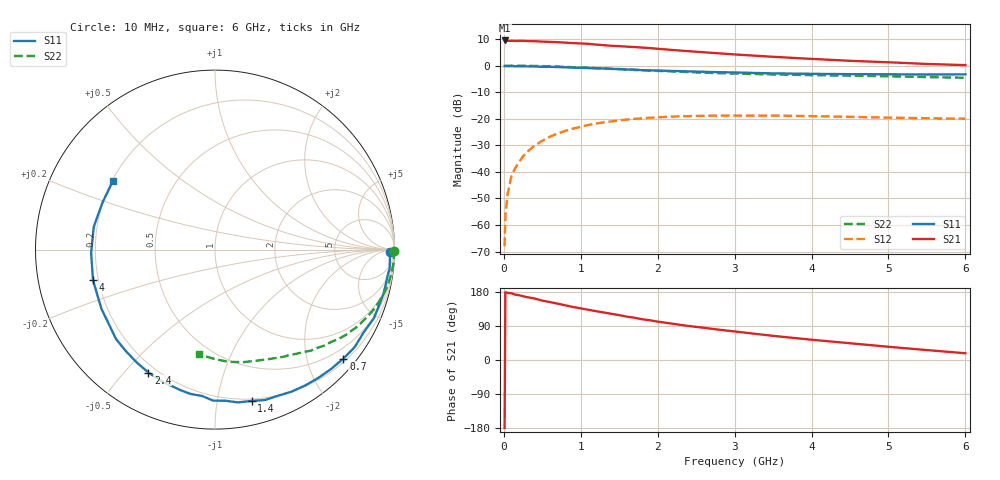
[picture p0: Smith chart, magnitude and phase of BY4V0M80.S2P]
! SIEMENS Small Signal Semiconductors
! BFY420
! Si NPN RF SIEGET Grounded Emitter Transistor in MICRO-X
! VCE = 4 V  IC = 0.8 mA
! Common Emitter S-Parameters:  October  1996
# GHz  S  MA  R  50
!  f  S11  S21  S12  S22
! GHz  MAG  ANG  MAG  ANG  MAG  ANG  MAG  ANG
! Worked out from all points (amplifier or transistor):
!   36 points, 10 MHz to 6 GHz, reference 50 ohm
!   highest |S21| = 9.5 dB at 10 MHz (marker M1)
!   |S21| within 3 dB of that: start of sweep to 1.947 GHz
!   unconditionally stable (mu >= 1): 4.579 GHz to end of sweep
!   at 250 MHz: K = 0.03, MSG = 21.7 dB, |S12| = -34.2 dB
!   at 1.4 GHz: K = 0.17, MSG = 14.2 dB, |S12| = -21.0 dB
!   at 6 GHz: K = 1.39, MAG = 6.4 dB, |S12| = -20.0 dB
!   S11 on the Smith chart (normalised r, x): 10 MHz: 63, -38; 700 MHz: 0.27, -2.70; 1.4 GHz: 0.18, -1.25; 2.4 GHz: 0.17, -0.58; 4 GHz: 0.18, -0.12; 6 GHz: 0.20, +0.29
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0.01  0.9771 -0.8  2.974 -179.4  0.0004 77.2  0.9998 -0.3
0.02  0.9761 -1.4  2.964 178.8  0.0015 88.6  0.9967 -0.5
0.05  0.9758 -3.2  2.921 177.2  0.0039 88.3  0.9983 -1.3
0.1  0.9788 -6.2  2.93 175.8  0.0085 86.4  0.9976 -2.6
0.15  0.9719 -8.9  2.913 172.4  0.0119 80.9  0.9961 -4.0
0.2  0.9709 -11.8  2.92 170.9  0.0155 82.4  0.9962 -5.1
0.3  0.9672 -17.3  2.898 166.0  0.0236 78.7  0.9911 -7.8
0.4  0.9643 -23.3  2.877 162.2  0.0312 76.1  0.9855 -10.4
0.5  0.9482 -29.0  2.828 156.7  0.0385 72.7  0.9784 -12.9
0.7  0.9384 -40.3  2.759 148.6  0.0528 65.6  0.9585 -17.8
0.9  0.9178 -51.2  2.652 139.8  0.0653 58.8  0.9344 -22.5
1.1  0.8988 -61.8  2.568 132.5  0.0764 53.0  0.9086 -27.0
1.4  0.8673 -76.4  2.356 121.8  0.0892 44.6  0.8711 -33.0
1.8  0.8185 -95.1  2.184 107.5  0.1019 34.7  0.8171 -40.0
2.2  0.7927 -111.4  1.966 95.5  0.1098 26.3  0.7767 -46.4
2.4  0.7791 -118.4  1.868 89.8  0.1121 23.1  0.7532 -49.4
2.8  0.7518 -131.8  1.702 79.9  0.1145 16.7  0.7195 -54.7
3.5  0.7135 -152.5  1.465 63.7  0.1147 8.7  0.6818 -63.3
4  0.7006 -166.0  1.338 53.5  0.112 4.5  0.6612 -69.4
4.5  0.6905 -178.4  1.231 44.2  0.1086 1.5  0.6466 -75.9
5.5  0.6795 157.5  1.074 26.2  0.1023 0.1  0.6086 -90.5
6  0.6849 146.3  1.022 17.8  0.1 1.5  0.5909 -98.7
